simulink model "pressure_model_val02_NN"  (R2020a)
settings: Solver=VariableStepAuto  StartTime=0.0  StopTime=tfin  RelTol=1e-3
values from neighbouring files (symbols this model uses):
  Ts = 5    [sisopres.m]
undefined symbols (not defined in the file or in its folder): magnitude
libraries: neural x10

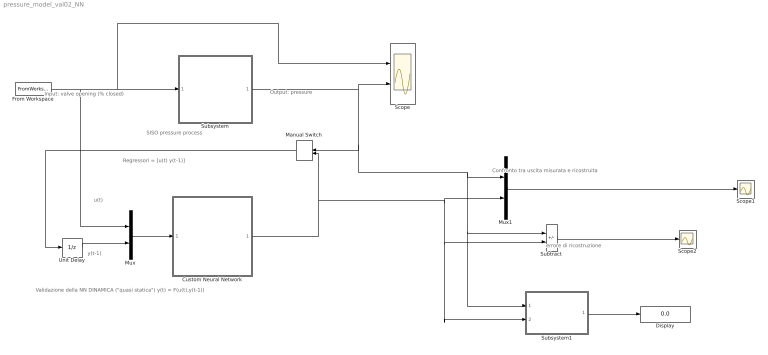
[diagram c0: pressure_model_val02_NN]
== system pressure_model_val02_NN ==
  note: Confronto tra uscita misurata e ricostruita
  note: Regressori = [u(t) y(t-1)]
  note: y(t-1)
  note: u(t)
  note: Validazione della NN DINAMICA ("quasi statica") y(t) = F(u(t),y(t-1))
  note: Output: pressure
  note: Input: valve opening (% closed)
  note: SISO pressure process
  note: errore di ricostruzione
  Custom Neural Network : Subsystem
      mask help: Custom Neural Network
  Display : Display
  From Workspace : FromWorkspace  VariableName=[tsim U]  SampleTime=Ts
  Manual Switch : ManualSwitch
  Mux : Mux  Inputs=2
  Mux1 : Mux  Inputs=2
  Scope : Scope  NumInputPorts=2
  Scope1 : Scope
  Scope2 : Scope
  Subsystem : Subsystem
  Subsystem1 : Subsystem
  Subtract : Sum  Inputs=+-
  Unit Delay : UnitDelay  SampleTime=Ts  HasFrameUpgradeWarning=on
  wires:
  From Workspace/1 -> Mux/1, Scope/1, Subsystem/1(u)
  Mux/1 -> Custom Neural Network/1(Input)
  Subsystem1/1(VAF%) -> Display/1
  Subtract/1 -> Scope2/1
  Subsystem/1(y) -> Manual Switch/1, Subsystem1/1(y_mis), Subtract/1, Mux1/1, Scope/2
  Custom Neural Network/1(Output) -> Manual Switch/2, Subsystem1/2(y_prev), Subtract/2, Mux1/2
  Mux1/1 -> Scope1/1
  Manual Switch/1 -> Unit Delay/1
  Unit Delay/1 -> Mux/2

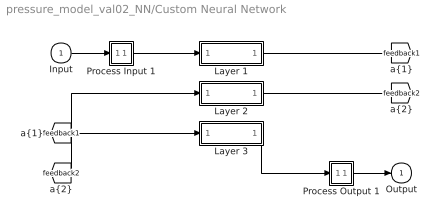
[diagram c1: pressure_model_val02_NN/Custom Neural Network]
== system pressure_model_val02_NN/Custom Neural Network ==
  Input : Inport  PortDimensions=2  SampleTime=5
  Layer 1 : Subsystem
  Layer 2 : Subsystem
  Layer 3 : Subsystem
  Process Input 1 : Subsystem
  Process Output 1 : Subsystem
  Output : Outport  InitialOutput=0
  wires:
  Input/1 -> Process Input 1/1(x)
  Process Output 1/1(y) -> Output/1
  Process Input 1/1(p) -> Layer 1/1("p{1}")
  Layer 1/1("a{1}") -> [feedback1]
  [feedback1] -> Layer 2/1("a{1} ")
  Layer 2/1("a{2}") -> [feedback2]
  [feedback2] -> Layer 3/1("a{2} ")
  Layer 3/1("a{3}") -> Process Output 1/1(a)

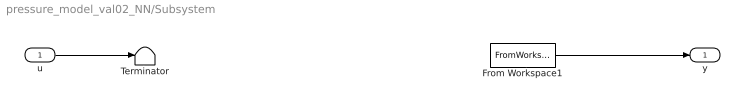
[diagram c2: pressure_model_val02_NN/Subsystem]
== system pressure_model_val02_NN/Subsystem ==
  u : Inport
  From Workspace1 : FromWorkspace  VariableName=[tsim Y]  SampleTime=Ts
  Terminator : Terminator
  y : Outport
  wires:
  From Workspace1/1 -> y/1
  u/1 -> Terminator/1

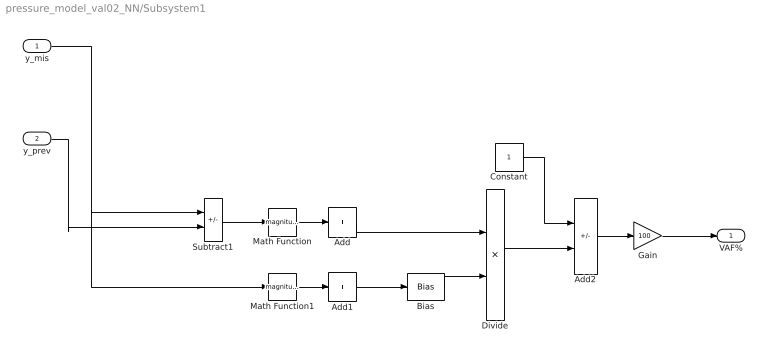
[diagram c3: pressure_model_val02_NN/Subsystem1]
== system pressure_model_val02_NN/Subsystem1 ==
  y_mis : Inport
  y_prev : Inport  Port=2
  Add : Sum  Inputs=+
  Add1 : Sum  Inputs=+
  Add2 : Sum  Inputs=+-
  Bias : Bias  Bias=1e-7
  Constant : Constant
  Divide : Product  Inputs=*/
  Gain : Gain  Gain=100
  Math Function : Math  Operator=magnitude^2
  Math Function1 : Math  Operator=magnitude^2
  Subtract1 : Sum  Inputs=+-
  VAF% : Outport
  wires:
  Add2/1 -> Gain/1
  Math Function/1 -> Add/1
  Bias/1 -> Divide/2
  y_mis/1 -> Math Function1/1, Subtract1/1
  Add1/1 -> Bias/1
  Math Function1/1 -> Add1/1
  Subtract1/1 -> Math Function/1
  Constant/1 -> Add2/1
  Divide/1 -> Add2/2
  Add/1 -> Divide/1
  y_prev/1 -> Subtract1/2
  Gain/1 -> VAF%/1

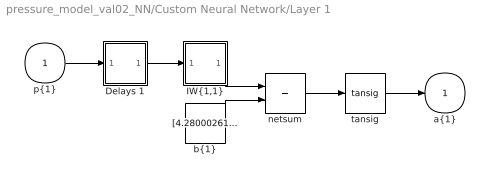
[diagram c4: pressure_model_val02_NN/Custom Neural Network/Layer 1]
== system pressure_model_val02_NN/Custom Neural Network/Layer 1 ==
  "p{1}" : Inport  PortDimensions=2  SampleTime=5
  Delays 1 : Subsystem
  "IW{1,1}" : Subsystem
  "b{1}" : Constant  Value=[4.2800026159692965421754706767387688159942626953125;-2.95042700888907827305729369982145726680755615234375]
  netsum : Sum  Inputs=2  InputSameDT=on  SaturateOnIntegerOverflow=on
  tansig : neural/Transfer Functions/tansig
  "a{1}" : Outport  InitialOutput=[0;0]
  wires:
  "p{1}"/1 -> Delays 1/1("p{1}")
  Delays 1/1("pd{1,1}") -> "IW{1,1}"/1("pd{1,1}")
  "IW{1,1}"/1("iz{1,1}") -> netsum/1
  "b{1}"/1 -> netsum/2
  netsum/1 -> tansig/1
  tansig/1 -> "a{1}"/1

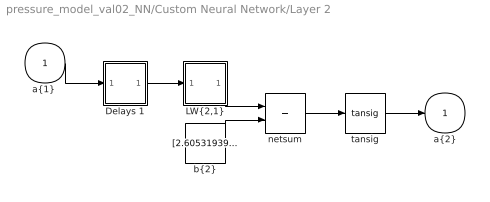
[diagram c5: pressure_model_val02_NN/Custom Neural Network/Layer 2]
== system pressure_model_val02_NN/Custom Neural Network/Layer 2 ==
  "a{1} " : Inport  PortDimensions=2  SampleTime=5
  Delays 1 : Subsystem
  "LW{2,1}" : Subsystem
  "b{2}" : Constant  Value=[2.605319396477325799565960551262833178043365478515625;-1.6147732448315952336059808658319525420665740966796875;1.027112978129435472141040008864365518093109130859375;-3.110517669286632980174545082263648509979248046875]
  netsum : Sum  Inputs=2  InputSameDT=on  SaturateOnIntegerOverflow=on
  tansig : neural/Transfer Functions/tansig
  "a{2}" : Outport  InitialOutput=[0;0;0;0]
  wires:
  "a{1} "/1 -> Delays 1/1("p{2}")
  Delays 1/1("pd{2,1}") -> "LW{2,1}"/1("ad{2,1}")
  "LW{2,1}"/1("lz{2,1}") -> netsum/1
  "b{2}"/1 -> netsum/2
  netsum/1 -> tansig/1
  tansig/1 -> "a{2}"/1

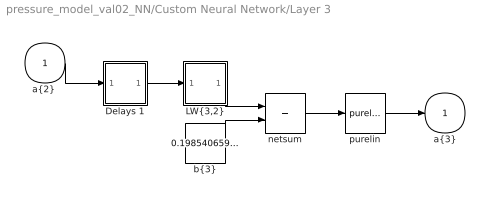
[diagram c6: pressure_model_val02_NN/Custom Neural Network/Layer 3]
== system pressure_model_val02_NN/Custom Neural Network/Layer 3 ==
  "a{2} " : Inport  PortDimensions=4  SampleTime=5
  Delays 1 : Subsystem
  "LW{3,2}" : Subsystem
  "b{3}" : Constant  Value=0.1985406591074303228605657523075933568179607391357421875
  netsum : Sum  Inputs=2  InputSameDT=on  SaturateOnIntegerOverflow=on
  purelin : neural/Transfer Functions/purelin
  "a{3}" : Outport  InitialOutput=0
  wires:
  "a{2} "/1 -> Delays 1/1("p{3}")
  Delays 1/1("pd{3,2}") -> "LW{3,2}"/1("ad{3,2}")
  "LW{3,2}"/1("lz{3,2}") -> netsum/1
  "b{3}"/1 -> netsum/2
  netsum/1 -> purelin/1
  purelin/1 -> "a{3}"/1

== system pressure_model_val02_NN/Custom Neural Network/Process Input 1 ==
  x : Inport  PortDimensions=2  SampleTime=5
  p : Outport  PortDimensions=2  SampleTime=5
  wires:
  x/1 -> p/1

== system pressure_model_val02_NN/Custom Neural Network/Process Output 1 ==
  a : Inport  PortDimensions=1  SampleTime=5
  y : Outport  PortDimensions=1  SampleTime=5
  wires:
  a/1 -> y/1

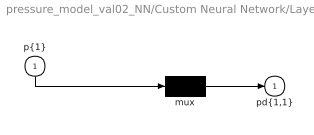
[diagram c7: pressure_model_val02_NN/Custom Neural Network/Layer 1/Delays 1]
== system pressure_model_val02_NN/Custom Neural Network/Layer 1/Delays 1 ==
  "p{1}" : Inport  PortDimensions=2  SampleTime=5
  mux : Mux  Inputs=1
  "pd{1,1}" : Outport
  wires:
  "p{1}"/1 -> mux/1
  mux/1 -> "pd{1,1}"/1

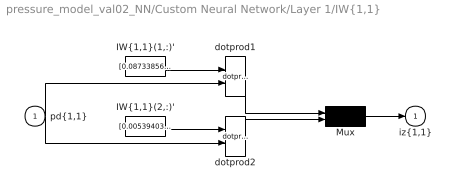
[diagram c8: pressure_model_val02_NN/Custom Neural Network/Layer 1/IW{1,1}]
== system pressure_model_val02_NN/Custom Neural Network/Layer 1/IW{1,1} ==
  "pd{1,1}" : Inport  PortDimensions=2  SampleTime=5
  "IW{1,1}(1,:)'" : Constant  Value=[0.08733856015114012383282471319034812040627002716064453125;1.440870717699436642789123652619309723377227783203125]
  "IW{1,1}(2,:)'" : Constant  Value=[0.005394030780961323566502496618113582371734082698822021484375;1.76606037871800936045474372804164886474609375]
  Mux : Mux  Inputs=2
  dotprod1 : neural/Weight Functions/dotprod
  dotprod2 : neural/Weight Functions/dotprod
  "iz{1,1}" : Outport
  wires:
  "IW{1,1}(1,:)'"/1 -> dotprod1/1
  "pd{1,1}"/1 -> dotprod1/2, dotprod2/2
  dotprod1/1 -> Mux/1
  "IW{1,1}(2,:)'"/1 -> dotprod2/1
  dotprod2/1 -> Mux/2
  Mux/1 -> "iz{1,1}"/1

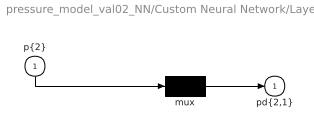
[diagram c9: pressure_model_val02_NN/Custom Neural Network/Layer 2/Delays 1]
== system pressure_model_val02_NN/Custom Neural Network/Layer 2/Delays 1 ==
  "p{2}" : Inport  PortDimensions=2  SampleTime=5
  mux : Mux  Inputs=1
  "pd{2,1}" : Outport
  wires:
  "p{2}"/1 -> mux/1
  mux/1 -> "pd{2,1}"/1

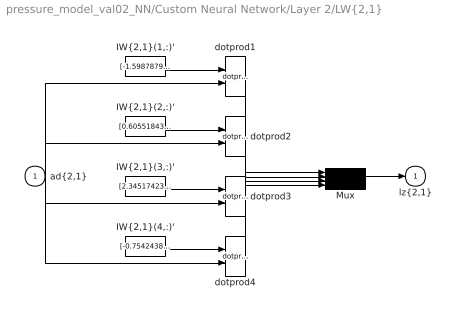
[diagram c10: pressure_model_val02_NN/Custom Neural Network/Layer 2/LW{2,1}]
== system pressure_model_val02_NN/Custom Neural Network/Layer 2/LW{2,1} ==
  "ad{2,1}" : Inport  PortDimensions=2  SampleTime=5
  "IW{2,1}(1,:)'" : Constant  Value=[-1.598787913745928879194480032310821115970611572265625;2.941702415189601627076854128972627222537994384765625]
  "IW{2,1}(2,:)'" : Constant  Value=[0.605518432022325470143186976201832294464111328125;1.4708738899425111146257449945551343262195587158203125]
  "IW{2,1}(3,:)'" : Constant  Value=[2.345174233668651186945908193592913448810577392578125;1.6226321967131436263542809683713130652904510498046875]
  "IW{2,1}(4,:)'" : Constant  Value=[-0.75424387430973183210625165884266607463359832763671875;-2.369365708245438018053619089187122881412506103515625]
  Mux : Mux
  dotprod{1..4} (4 alike) : neural/Weight Functions/dotprod
  "lz{2,1}" : Outport
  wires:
  "IW{2,1}(1,:)'"/1 -> dotprod1/1
  "ad{2,1}"/1 -> dotprod1/2, dotprod2/2, dotprod3/2, dotprod4/2
  dotprod1/1 -> Mux/1
  "IW{2,1}(2,:)'"/1 -> dotprod2/1
  dotprod2/1 -> Mux/2
  "IW{2,1}(3,:)'"/1 -> dotprod3/1
  dotprod3/1 -> Mux/3
  "IW{2,1}(4,:)'"/1 -> dotprod4/1
  dotprod4/1 -> Mux/4
  Mux/1 -> "lz{2,1}"/1

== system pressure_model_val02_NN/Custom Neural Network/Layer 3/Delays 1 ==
  "p{3}" : Inport  PortDimensions=4  SampleTime=5
  mux : Mux  Inputs=1
  "pd{3,2}" : Outport
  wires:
  "p{3}"/1 -> mux/1
  mux/1 -> "pd{3,2}"/1

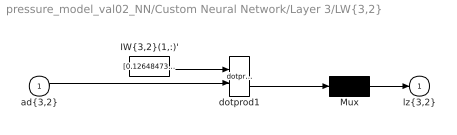
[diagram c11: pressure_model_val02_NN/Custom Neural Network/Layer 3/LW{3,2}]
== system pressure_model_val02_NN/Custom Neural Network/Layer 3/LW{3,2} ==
  "ad{3,2}" : Inport  PortDimensions=4  SampleTime=5
  "IW{3,2}(1,:)'" : Constant  Value=[0.126484739837429083220143866128637455403804779052734375;0.53860805638055209154657632097951136529445648193359375;0.97274124735805778119157594119315035641193389892578125;-0.59345495867598085926175599524867720901966094970703125]
  Mux : Mux  Inputs=1
  dotprod1 : neural/Weight Functions/dotprod
  "lz{3,2}" : Outport
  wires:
  "IW{3,2}(1,:)'"/1 -> dotprod1/1
  "ad{3,2}"/1 -> dotprod1/2
  dotprod1/1 -> Mux/1
  Mux/1 -> "lz{3,2}"/1
